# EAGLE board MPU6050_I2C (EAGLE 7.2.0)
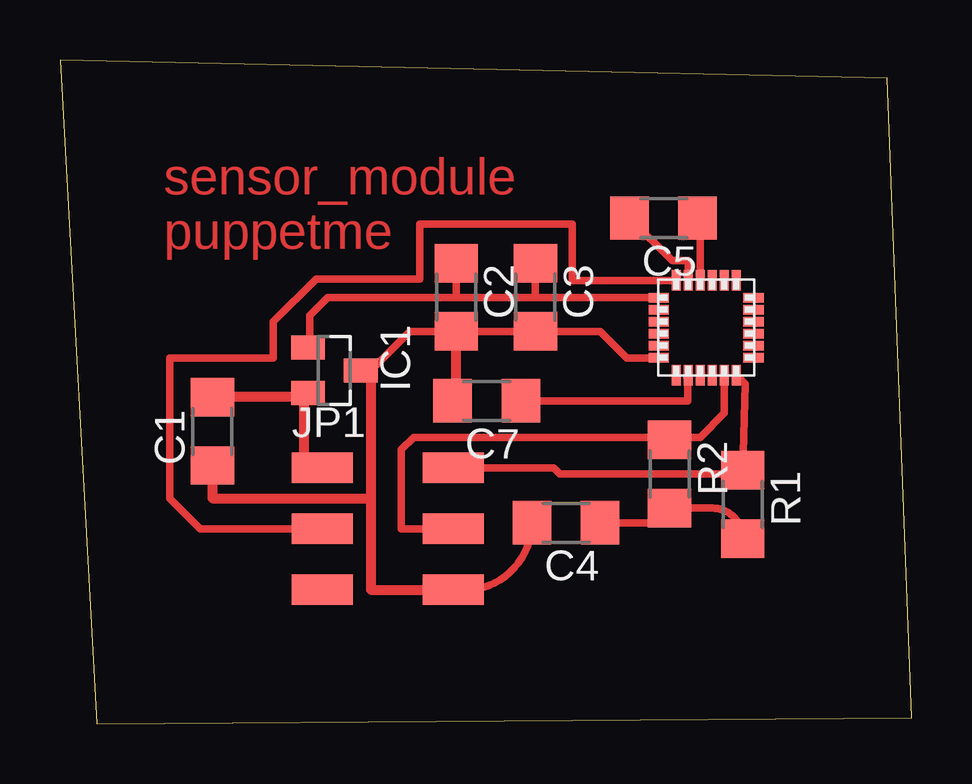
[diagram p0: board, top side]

Size 35.48 x 27.68 mm. Coordinates in mm from the lower left corner, seen from the top.
Outline: 1.52,0 35.48,0.25 34.47,26.91 0,27.68 1.52,0
Copper layers (1*16): Top 0.035mm / dielectric 1.5mm / Bottom 0.035mm
Design rules "default": minimum track width 10mil, minimum drill 24mil, track to track 8mil, track to pad 8mil, pad to pad 8mil, via to via 8mil, smd to smd 8mil, copper to edge 40mil, drill to drill 8mil, minimum pad ring 10mil, minimum via ring 8mil, stop-mask expansion 4mil, vias tented up to drill 0mil, thermal gap 10mil

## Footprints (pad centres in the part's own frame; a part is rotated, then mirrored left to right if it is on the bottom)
1206 = smd 1.6 x 1.803: 1 -1.422,0; 2 1.422,0
SOT23 = smd 1 x 1.4: 1 -0.95,-1.1; 2 0.95,-1.1; 3 0,1.1
2X03SMD = smd 2.54 x 1.27: 1 -2.54,2.54; 2 2.92,2.54; 3 -2.54,0; 4 2.92,0; 5 -2.54,-2.54; 6 2.92,-2.54
QFN.24.4X4 = smd 0.85 x 0.38: 1 -1.975,1.25; 2 -1.975,0.75; 3 -1.975,0.25; 4 -1.975,-0.25; 5 -1.975,-0.75; 6 -1.975,-1.25; 13 1.975,-1.25; 14 1.975,-0.75; 15 1.975,-0.25; 16 1.975,0.25; 17 1.975,0.75; 18 1.975,1.25 | smd 0.38 x 0.85: 7 -1.25,-1.975; 8 -0.75,-1.975; 9 -0.25,-1.975; 10 0.25,-1.975; 11 0.75,-1.975; 12 1.25,-1.975; 19 1.25,1.975; 20 0.75,1.975; 21 0.25,1.975; 22 -0.25,1.975; 23 -0.75,1.975; 24 -1.25,1.975

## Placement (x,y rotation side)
C1  4.7uF  [1206]  6.35,12.19 90 top
C2  10uF  [1206]  16.51,17.78 270 top
C3  0.1uF  [1206]  19.81,17.78 270 top
C4  0.01uF  [1206]  21.08,8.38 180 top
C5  0.1uF  [1206]  25.15,21.08 180 top
C7  2.2nF  [1206]  17.78,13.46 180 top
IC1  [SOT23]  11.43,14.73 270 top
JP1  [2X03SMD]  13.46,8.13 0 top
R1  [1206]  28.45,9.14 270 top
R2  [1206]  25.4,10.41 270 top
U$1  MPU-6050  [QFN.24.4X4]  26.92,16.51 180 top

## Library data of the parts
C1-C5 C7 IC1 R1 R2 = ng
JP1 = fab
U$1 = invensense

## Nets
CPOUT: C7.1 U$1.20
GND: C1.1 C2.2 C3.2 C4.2 C7.2 IC1.3 JP1.6 U$1.18
INT: JP1.3 U$1.12
N$1: C5.1 U$1.10
N$2: C5.2 U$1.11
SCL: JP1.4 R2.1 U$1.23
SDA: JP1.2 R1.1 U$1.24
VCC_5V: C1.2 IC1.2 JP1.1
VDD: C4.1 R1.2 R2.2
VLOGIC: C2.1 C3.1 IC1.1 U$1.13

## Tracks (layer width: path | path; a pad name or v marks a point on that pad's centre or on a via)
CPOUT
  Top 0.305: 26.16,14.48 26.16,13.46 C7.1
  Top 0.406: U$1.20 26.16,14.52 26.16,14.48
GND
  Top 0.305: 12.95,14.73 14.58,16.36 C2.2 C3.2 22.5,16.36 23.62,15.24 24.93,15.24 U$1.18 | JP1.6 16.87,5.59 arc90 C4.2
  Top 0.406: 12.95,9.4 12.95,14.73 IC1.3 | 12.95,9.4 12.95,5.59 JP1.6 | C7.2 16.51,13.61 C2.2 | C1.1 6.35,9.4 12.95,9.4
INT
  Top 0.305: U$1.12 21.34,18.48 21.34,20.83 14.99,20.83 14.99,18.54 10.67,18.54 8.89,16.76 8.89,15.24 4.57,15.24 4.57,9.4 5.84,8.13 JP1.3
N$1
  Top 0.305: U$1.10 26.67,21.08 C5.1
N$2
  Top 0.305: U$1.11 26.17,19.3 25.5,19.3 C5.2
SCL
  Top 0.305: U$1.23 27.67,12.97 27.69,12.95 26.67,11.94 25.5,11.94 R2.1 25.3,11.94 14.73,11.94 14.22,11.43 14.22,8.13 JP1.4
SDA
  Top 0.305: U$1.24 28.55,14.16 R1.1 28.3,10.41 20.83,10.41 20.57,10.67 JP1.2
VCC_5V
  Top 0.406: 10.16,13.72 10.16,13.78 IC1.2 10.26,13.72 10.16,13.72 | 10.16,13.72 10.16,10.67 JP1.1 | 10.16,13.72 10.06,13.61 C1.2
VDD
  Top 0.305: C4.1 24.79,8.38 arc90 R2.2 27.18,8.99 arc-90 R1.2
VLOGIC
  Top 0.305: IC1.1 10.41,15.68 10.41,17.02 11.16,17.76 16.51,17.76 | 19.81,17.76 16.76,17.76 16.51,17.76 | 19.81,17.76 U$1.13 | C3.1 19.81,17.76 | C2.1 16.51,17.76

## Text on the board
Top: sensor_module / puppetme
